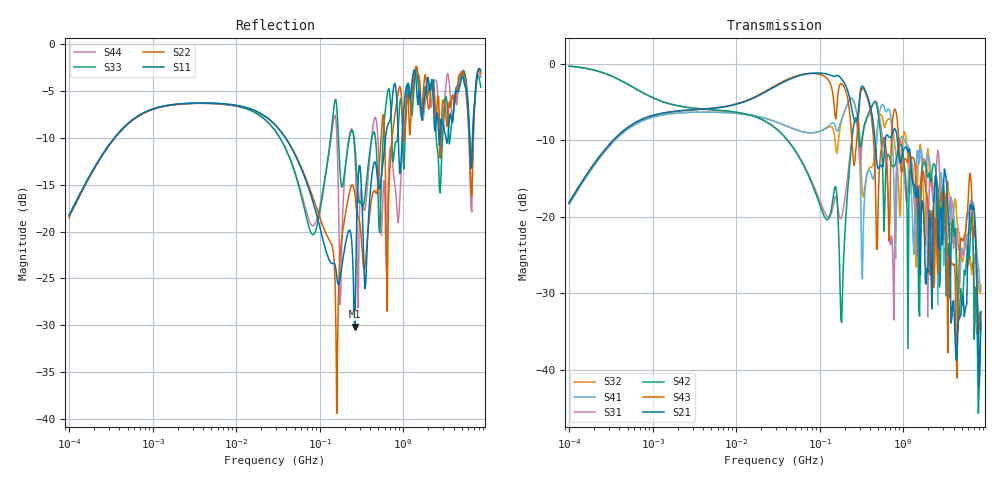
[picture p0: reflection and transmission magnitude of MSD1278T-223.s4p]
# MHz S MA R 50
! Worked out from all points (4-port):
!   498 points, 100 kHz to 8.5 GHz, reference 50 ohm
!   strongest paths, dB at 100 kHz, 1.698 MHz, 29.49 MHz, 500.7 MHz, 8.5 GHz:
!     S21: -18.2, -6.2, -2.9, -13.7, -32.4
!     S43: -18.1, -6.3, -2.8, -18.3, -32.6
!     S42: -0.3, -5.3, -8.4, -6.5, -33.9
!     S31: -0.3, -5.3, -8.4, -5.8, -34.6
!     S41: -18.3, -6.5, -7.5, -7.7, -29.7
!     S32: -18.3, -6.5, -7.5, -7.5, -29.0
!   lowest |S11| = -30.2 dB at 264.1 MHz (marker M1), VSWR 1.06, Z = 47 + j0.184 ohm
!   |S11| at or under -10 dB: 38.97 MHz to 613.1 MHz (574.1 MHz wide, 176 % of centre); 3.251 GHz to 3.432 GHz (180.6 MHz wide, 5.4 % of centre); 6.224 GHz to 6.808 GHz (583.6 MHz wide, 8.96 % of centre)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
0.1  0.1225 73.2  0.1237 73.9  0.9672 -7.1  0.1211 -106.5
     0.1237 73.9  0.1188 73.8  0.1212 -106.5  0.9678 -7.1
     0.9672 -7.1  0.1212 -106.5  0.1214 73.8  0.1243 73.6
     0.1211 -106.5  0.9678 -7.1  0.1243 73.6  0.1222 74.1
183.289  0.06462 -2.3  0.7962 -52.2  0.1004 101.1  0.4383 25.5
         0.7962 -52.2  0.09164 10.3  0.428 35.6  0.02038 87.9
         0.1004 101.1  0.428 35.6  0.173 -37.4  0.7432 -52.1
         0.4383 25.5  0.02038 87.9  0.7432 -52.1  0.08364 20.6
264.1375  0.03101 176.4  0.4236 -60.4  0.4223 38.8  0.5381 -47.4
          0.4236 -60.4  0.1569 -109.1  0.5349 -35.3  0.4342 50.7
          0.4223 38.8  0.5349 -35.3  0.286 -108.7  0.2352 -46.3
          0.5381 -47.4  0.4342 50.7  0.2352 -46.3  0.2514 -81.2
1306.515  0.6904 -123.4  0.1649 172.2  0.181 -139.5  0.07389 90.6
          0.1649 172.2  0.5922 -107.6  0.2027 -169.8  0.1653 -173.7
          0.181 -139.5  0.2027 -169.8  0.4855 -117.8  0.2451 -163.3
          0.07389 90.6  0.1653 -173.7  0.2451 -163.3  0.6752 -114.0
3183.684  0.3353 42.8  0.1934 49.3  0.07222 -3.0  0.06278 30.0
          0.1934 49.3  0.4669 42.3  0.0911 25.6  0.079 -65.8
          0.07222 -3.0  0.0911 25.6  0.5078 60.0  0.1347 13.8
          0.06278 30.0  0.079 -65.8  0.1347 13.8  0.5565 74.1
4284.188  0.5641 -51.1  0.01154 60.7  0.07584 -89.6  0.06265 -97.9
          0.01154 60.7  0.5429 -57.2  0.1208 -93.0  0.06889 -118.6
          0.07584 -89.6  0.1208 -93.0  0.5864 -58.8  0.01565 177.7
          0.06265 -97.9  0.06889 -118.6  0.01565 177.7  0.5125 -65.3
8500  0.7237 -54.4  0.02402 -34.7  0.01869 -76.6  0.03278 -162.7
      0.02402 -34.7  0.6989 -63.9  0.03541 153.2  0.02017 -65.2
      0.01869 -76.6  0.03541 153.2  0.5911 -61.2  0.02355 -78.5
      0.03278 -162.7  0.02017 -65.2  0.02355 -78.5  0.6672 -57.1
